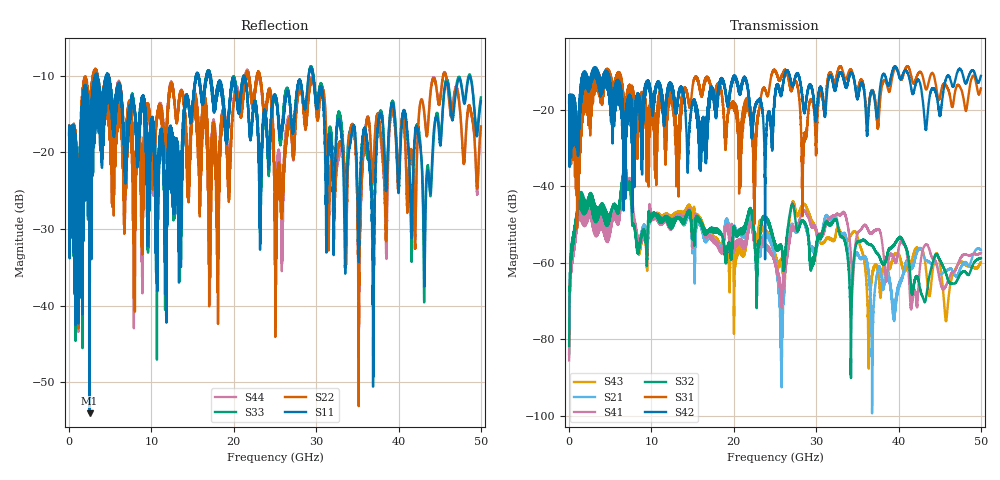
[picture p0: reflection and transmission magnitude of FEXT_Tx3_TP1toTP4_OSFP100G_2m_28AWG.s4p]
! Touchstone data
! Created: 27-Feb-2019 by IdEM 12 (12.1.0)
! COMMENTS
!  Created Wed Feb 27 12:03:36 2019
!  64 Port Network Data from SP1.SP block
!  freq  magS1_1  angS1_1  magS1_2  angS1_2  magS1_3  angS1_3  magS1_4  angS1_4
!  magS1_5  angS1_5  magS1_6  angS1_6  magS1_7  angS1_7  magS1_8  angS1_8
!  magS1_9  angS1_9  magS1_10  angS1_10  magS1_11  angS1_11  magS1_12  angS1_12
!  magS1_13  angS1_13  magS1_14  angS1_14  magS1_15  angS1_15  magS1_16  angS1_16
!  magS1_17  angS1_17  magS1_18  angS1_18  magS1_19  angS1_19  magS1_20  angS1_20
!  magS1_21  angS1_21  magS1_22  angS1_22  magS1_23  angS1_23  magS1_24  angS1_24
!  magS1_25  angS1_25  magS1_26  angS1_26  magS1_27  angS1_27  magS1_28  angS1_28
!  magS1_29  angS1_29  magS1_30  angS1_30  magS1_31  angS1_31  magS1_32  angS1_32
!  magS1_33  angS1_33  magS1_34  angS1_34  magS1_35  angS1_35  magS1_36  angS1_36
!  magS1_37  angS1_37  magS1_38  angS1_38  magS1_39  angS1_39  magS1_40  angS1_40
!  magS1_41  angS1_41  magS1_42  angS1_42  magS1_43  angS1_43  magS1_44  angS1_44
!  magS1_45  angS1_45  magS1_46  angS1_46  magS1_47  angS1_47  magS1_48  angS1_48
!  magS1_49  angS1_49  magS1_50  angS1_50  magS1_51  angS1_51  magS1_52  angS1_52
!  magS1_53  angS1_53  magS1_54  angS1_54  magS1_55  angS1_55  magS1_56  angS1_56
!  magS1_57  angS1_57  magS1_58  angS1_58  magS1_59  angS1_59  magS1_60  angS1_60
!  magS1_61  angS1_61  magS1_62  angS1_62  magS1_63  angS1_63  magS1_64  angS1_64
!  magS2_1  angS2_1  magS2_2  angS2_2  magS2_3  angS2_3  magS2_4  angS2_4
!  magS2_5  angS2_5  magS2_6  angS2_6  magS2_7  angS2_7  magS2_8  angS2_8
!  magS2_9  angS2_9  magS2_10  angS2_10  magS2_11  angS2_11  magS2_12  angS2_12
!  magS2_13  angS2_13  magS2_14  angS2_14  magS2_15  angS2_15  magS2_16  angS2_16
!  magS2_17  angS2_17  magS2_18  angS2_18  magS2_19  angS2_19  magS2_20  angS2_20
!  magS2_21  angS2_21  magS2_22  angS2_22  magS2_23  angS2_23  magS2_24  angS2_24
!  magS2_25  angS2_25  magS2_26  angS2_26  magS2_27  angS2_27  magS2_28  angS2_28
!  magS2_29  angS2_29  magS2_30  angS2_30  magS2_31  angS2_31  magS2_32  angS2_32
!  magS2_33  angS2_33  magS2_34  angS2_34  magS2_35  angS2_35  magS2_36  angS2_36
!  magS2_37  angS2_37  magS2_38  angS2_38  magS2_39  angS2_39  magS2_40  angS2_40
!  magS2_41  angS2_41  magS2_42  angS2_42  magS2_43  angS2_43  magS2_44  angS2_44
!  magS2_45  angS2_45  magS2_46  angS2_46  magS2_47  angS2_47  magS2_48  angS2_48
!  magS2_49  angS2_49  magS2_50  angS2_50  magS2_51  angS2_51  magS2_52  angS2_52
!  magS2_53  angS2_53  magS2_54  angS2_54  magS2_55  angS2_55  magS2_56  angS2_56
!  magS2_57  angS2_57  magS2_58  angS2_58  magS2_59  angS2_59  magS2_60  angS2_60
!  magS2_61  angS2_61  magS2_62  angS2_62  magS2_63  angS2_63  magS2_64  angS2_64
!  magS3_1  angS3_1  magS3_2  angS3_2  magS3_3  angS3_3  magS3_4  angS3_4
!  magS3_5  angS3_5  magS3_6  angS3_6  magS3_7  angS3_7  magS3_8  angS3_8
!  magS3_9  angS3_9  magS3_10  angS3_10  magS3_11  angS3_11  magS3_12  angS3_12
!  magS3_13  angS3_13  magS3_14  angS3_14  magS3_15  angS3_15  magS3_16  angS3_16
!  magS3_17  angS3_17  magS3_18  angS3_18  magS3_19  angS3_19  magS3_20  angS3_20
!  magS3_21  angS3_21  magS3_22  angS3_22  magS3_23  angS3_23  magS3_24  angS3_24
!  magS3_25  angS3_25  magS3_26  angS3_26  magS3_27  angS3_27  magS3_28  angS3_28
!  magS3_29  angS3_29  magS3_30  angS3_30  magS3_31  angS3_31  magS3_32  angS3_32
!  magS3_33  angS3_33  magS3_34  angS3_34  magS3_35  angS3_35  magS3_36  angS3_36
!  magS3_37  angS3_37  magS3_38  angS3_38  magS3_39  angS3_39  magS3_40  angS3_40
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# Hz S MA R 50
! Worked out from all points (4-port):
!   5000 points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, 10 MHz to 50 GHz, reference 50 ohm
!   strongest paths, dB at 10 MHz, 12.51 GHz, 25.01 GHz, 37.51 GHz, 50 GHz:
!     S42: -18.0, -14.4, -15.7, -20.1, -11.1
!     S31: -18.0, -16.4, -9.6, -24.1, -14.3
!     S32: -81.8, -49.7, -55.0, -57.8, -58.8
!     S41: -85.5, -49.3, -60.4, -51.2, -57.4
!     S21: -84.0, -49.5, -59.6, -61.7, -56.6
!     S43: -83.8, -48.6, -58.0, -62.2, -59.8
!   lowest |S11| = -54.1 dB at 2.49 GHz (marker M1), VSWR 1.00, Z = 49.8 + j0.0446 ohm
!   |S11| at or under -10 dB: 4.81 GHz to 15.41 GHz (10.6 GHz wide, 105 % of centre); 17.19 GHz to 29.09 GHz (11.9 GHz wide, 51.4 % of centre); 29.64 GHz to end of sweep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
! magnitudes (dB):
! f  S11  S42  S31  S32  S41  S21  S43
! 10 MHz  -17.7  -18.0  -18.0  -81.8  -85.5  -84.0  -83.8
! 2.49 GHz  -54.1  -14.3  -22.3  -44.2  -47.1  -45.9  -45.6
! 22.01 GHz  -17.9  -20.7  -22.7  -46.3  -50.1  -47.8  -49.7
! 25.76 GHz  -17.2  -15.4  -11.2  -56.0  -67.4  -76.9  -60.1
! 28.31 GHz  -12.0  -16.2  -45.3  -49.1  -46.7  -49.2  -44.9
! 36.83 GHz  -34.0  -15.0  -14.8  -55.6  -52.0  -84.5  -62.6
! 50 GHz  -13.3  -11.1  -14.3  -58.8  -57.4  -56.6  -59.8
